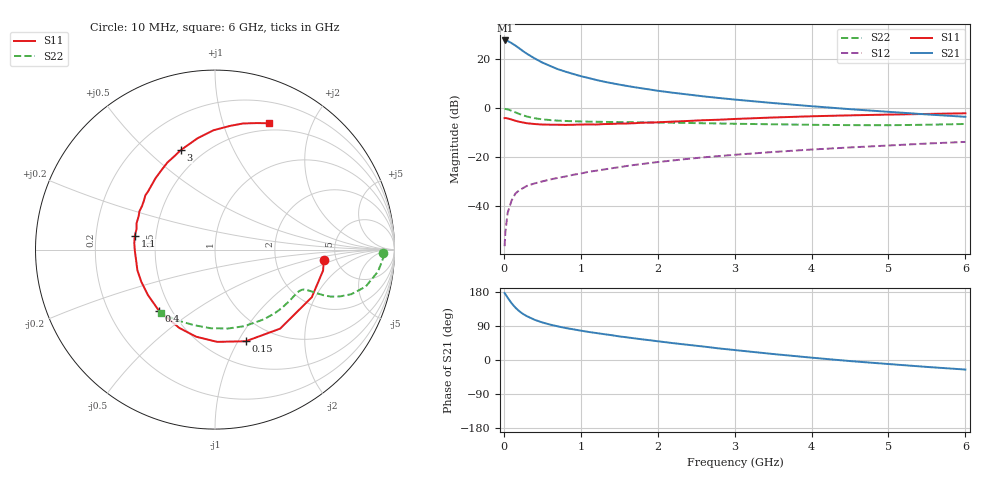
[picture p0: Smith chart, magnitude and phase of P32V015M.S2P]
! SIEMENS Small Signal Semiconductors
! BFP181
! Si NPN RF Bipolar Junction Transistor in SOT143
! VCE = 2 V  IC = 15 mA
! Common Emitter S-Parameters:  March  1996
# GHz  S  MA  R  50
!  f  S11  S21  S12  S22
! GHz  MAG  ANG  MAG  ANG  MAG  ANG  MAG  ANG
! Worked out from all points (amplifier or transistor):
!   36 points, 10 MHz to 6 GHz, reference 50 ohm
!   highest |S21| = 27.4 dB at 20 MHz (marker M1)
!   |S21| within 3 dB of that: start of sweep to 191.6 MHz
!   unconditionally stable (mu >= 1): start of sweep to 11.47 MHz; 537.7 MHz to end of sweep
!   at 250 MHz: K = 0.59, MSG = 27.9 dB, |S12| = -32.8 dB
!   at 1.4 GHz: K = 1.45, MAG = 13.4 dB, |S12| = -24.7 dB
!   at 6 GHz: K = 1.15, MAG = 2.8 dB, |S12| = -14.0 dB
!   S11 on the Smith chart (normalised r, x): 10 MHz: 3.98, -0.73; 150 MHz: 0.75, -1.08; 400 MHz: 0.43, -0.37; 1.1 GHz: 0.38, +0.07; 3 GHz: 0.38, +0.64; 6 GHz: 0.42, +1.43
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0.01  0.6092 -5.4  23.29 176.8  0.0015 83.4  0.9376 -1.3
0.02  0.6133 -11.0  23.32 173.9  0.0029 83.1  0.9379 -2.9
0.05  0.601 -26.2  22.71 164.2  0.0072 79.3  0.9167 -7.6
0.1  0.5707 -50.5  20.62 150.1  0.0127 67.0  0.8647 -13.8
0.15  0.5386 -71.4  18.34 138.2  0.0177 61.2  0.7994 -18.1
0.2  0.5143 -88.6  16.16 128.9  0.0207 56.3  0.7424 -20.6
0.25  0.4966 -102.2  14.12 121.4  0.0229 53.5  0.6957 -22.1
0.3  0.4796 -114.6  12.51 115.6  0.0254 51.4  0.6576 -22.8
0.4  0.4625 -132.3  10.05 106.1  0.0285 49.7  0.6066 -23.3
0.5  0.4514 -145.9  8.278 99.1  0.0313 48.9  0.5764 -23.5
0.6  0.448 -156.4  7.074 93.5  0.0342 49.6  0.5566 -23.8
0.7  0.4475 -165.1  6.079 88.8  0.0369 51.3  0.5427 -24.2
0.9  0.4464 -178.7  4.852 81.1  0.0427 51.7  0.5271 -25.6
1.1  0.4533 170.4  4.004 74.1  0.0491 53.1  0.5175 -27.6
1.3  0.4611 161.5  3.376 68.3  0.0547 53.2  0.5112 -30.1
1.5  0.472 153.2  2.941 62.3  0.0609 53.4  0.5068 -32.6
2.2  0.5179 129.7  2.005 44.5  0.0838 51.5  0.4905 -43.7
3  0.5862 109.0  1.458 26.3  0.1092 46.6  0.4676 -58.5
3.5  0.6279 98.9  1.237 15.8  0.1245 43.1  0.4566 -69.2
4.5  0.6946 83.0  0.928 -2.8  0.1541 35.2  0.4388 -93.2
5.5  0.7416 71.9  0.725 -18.3  0.185 27.5  0.447 -118.1
6  0.7655 66.9  0.649 -25.2  0.1998 22.9  0.4635 -130.2
